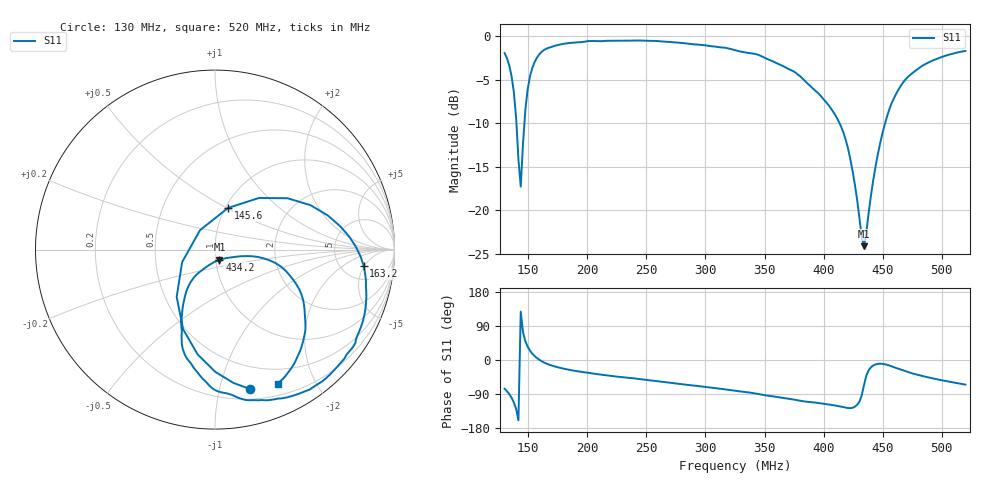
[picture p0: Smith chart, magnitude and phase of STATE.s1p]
!Agilent N9912A: A.05.34
!Date: Friday, 14 June 2013 16:35:32
!Model: N9912A
!Serial: MY50492702
!CABLE_LOSS: 0.000
!CABLE_NAME:
!VELOCITY_FACTOR: 1.000000000
!GPS Latitude:
!GPS Longitude:
!GPS TimeStamp: 0001-01-01 00:00:00Z
!GPS Seconds Since Last Read: 0
!CHECKSUM:1686277068
!Correction: S11(ON*)
!S1P File: Measurement: S11:
# Hz S DB R 50
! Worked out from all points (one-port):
!   201 points, 130 MHz to 520 MHz, reference 50 ohm
!   lowest |S11| = -24.1 dB at 434.2 MHz (marker M1), VSWR 1.13, Z = 52.2 - j5.95 ohm
!   |S11| at or under -10 dB: 140 MHz to 146.8 MHz (6.764 MHz wide, 4.72 % of centre); 413.5 MHz to 452 MHz (38.56 MHz wide, 8.91 % of centre)
!   S11 on the Smith chart (normalised r, x): 130 MHz: 0.29, -1.24; 145.6 MHz: 1.03, +0.51; 163.2 MHz: 8.09, -4.83; 434.2 MHz: 1.04, -0.12; 520 MHz: 0.33, -1.52
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1.3e8  -1.92 -75.8
1.3585e8  -4.55 -99.4
1.3975e8  -9.39 -129.0
1.417e8  -14.16 -159.2
1.4365e8  -17.29 127.6
1.456e8  -12.28 72.6
1.4755e8  -8.46 49.6
1.495e8  -6.11 35.3
1.534e8  -3.65 16.8
1.573e8  -2.47 5.4
1.6315e8  -1.58 -6.3
1.7875e8  -0.89 -22.0
2.041e8  -0.53 -35.4
2.275e8  -0.50 -44.6
2.7625e8  -0.71 -62.5
3.25e8  -1.58 -81.3
3.445e8  -2.12 -89.8
3.7375e8  -3.97 -103.7
4.069e8  -8.43 -118.6
4.1665e8  -11.03 -124.6
4.225e8  -14.04 -127.1
4.342e8  -24.15 -66.2
4.42e8  -16.56 -14.5
4.498e8  -11.15 -10.2
4.576e8  -7.69 -16.8
4.7125e8  -4.68 -31.8
4.927e8  -2.76 -48.7
5.2e8  -1.68 -65.0
